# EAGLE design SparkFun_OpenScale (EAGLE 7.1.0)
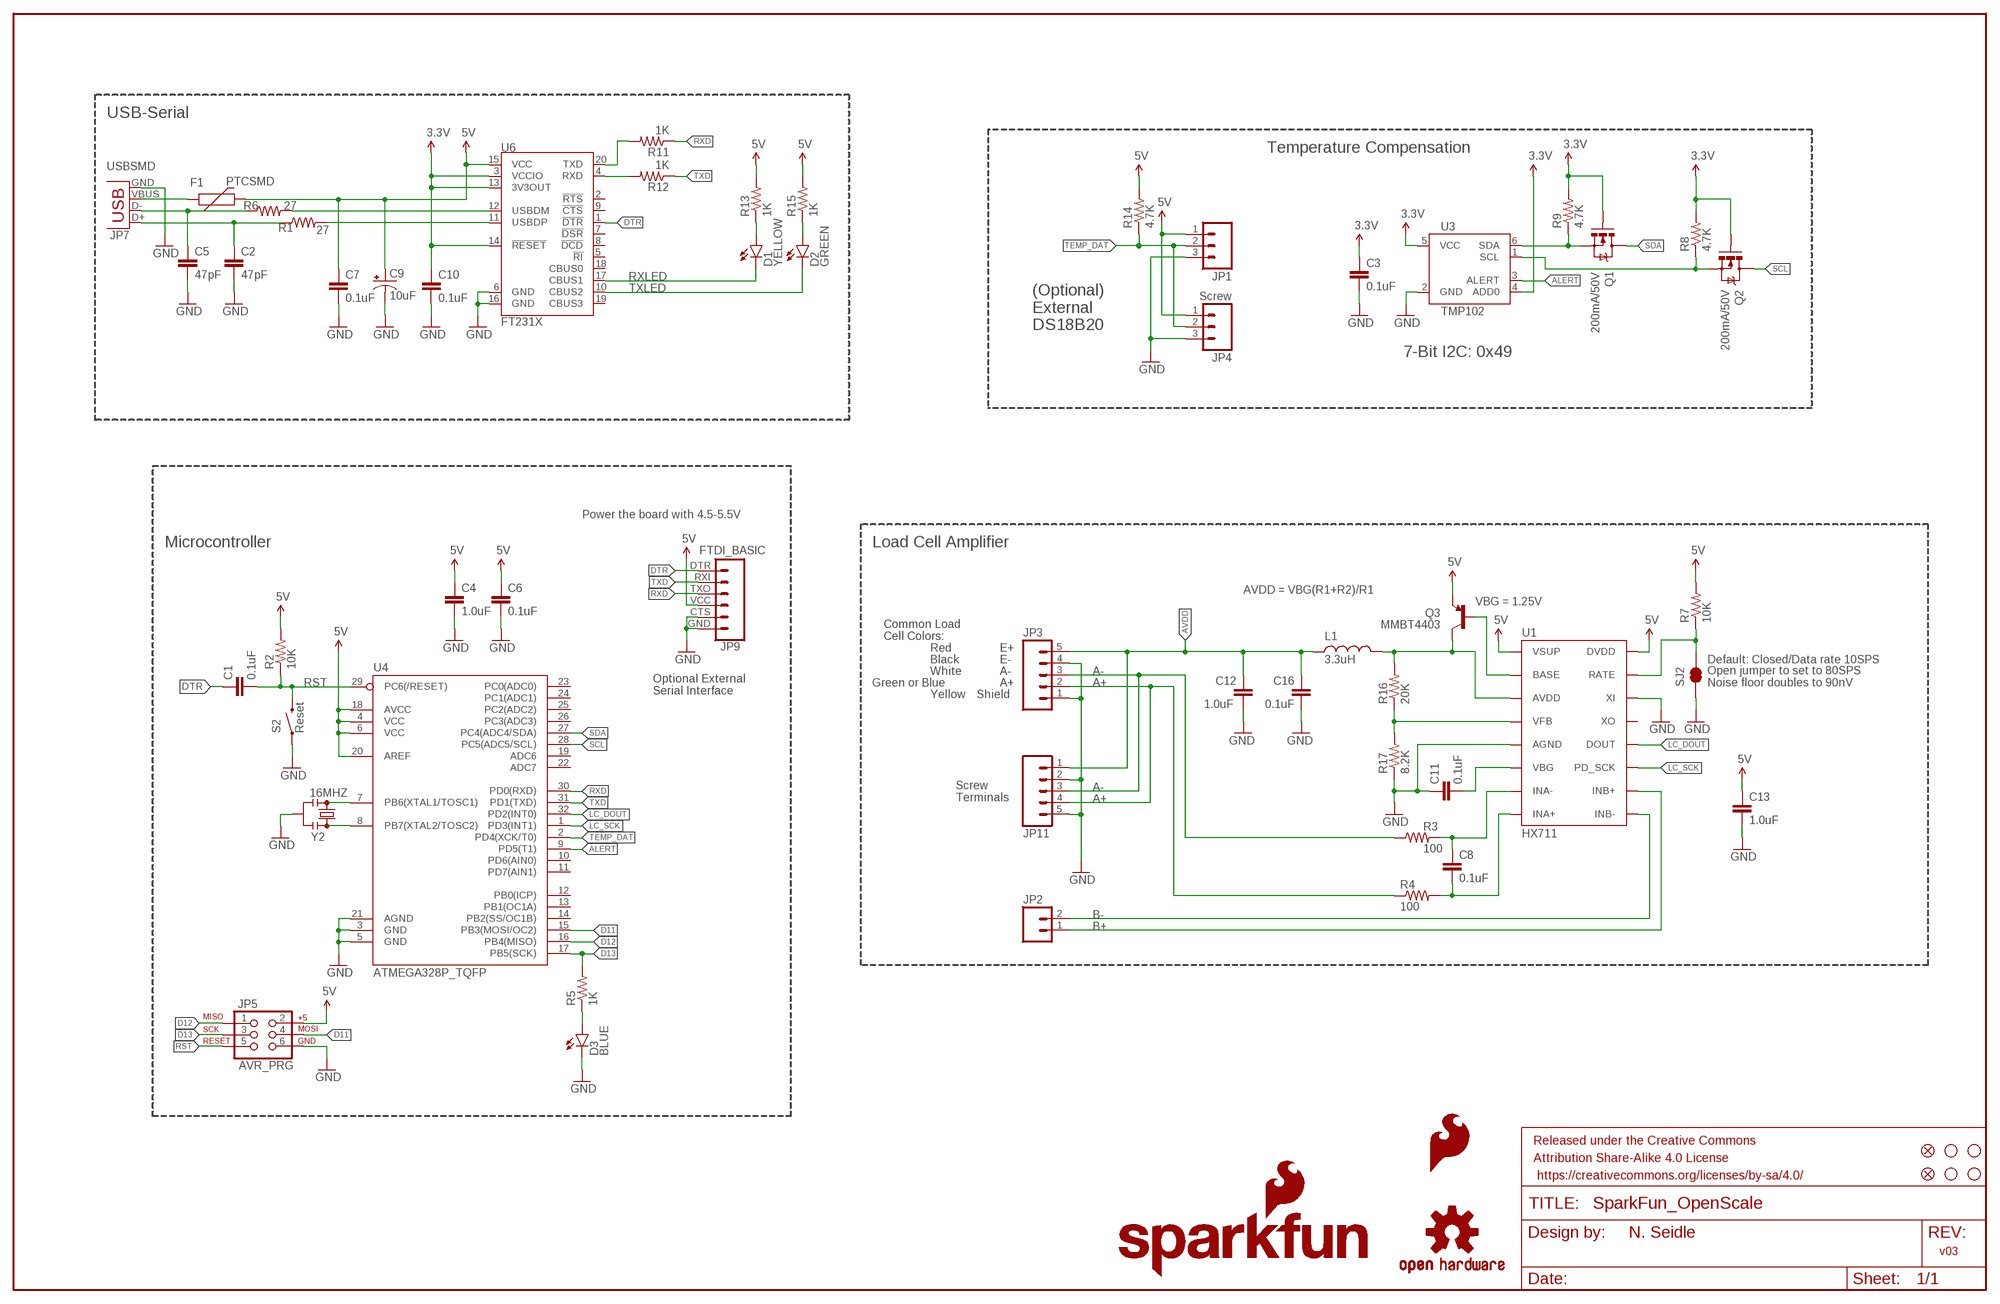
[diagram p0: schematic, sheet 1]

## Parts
C1  0.1uF  0.1UF-25V(+80/-20%)(0603)  [0603-CAP]
C2  47pF  47PF-50V-5%(0603)  [0603-CAP]
C3  0.1uF  0.1UF-25V(+80/-20%)(0603)  [0603-CAP]
C4  1.0uF  1.0UF-16V-10%(0603)  [0603-CAP]
C5  47pF  47PF-50V-5%(0603)  [0603-CAP]
C6  0.1uF  0.1UF-25V(+80/-20%)(0603)  [0603-CAP]
C7  0.1uF  0.1UF-25V(+80/-20%)(0603)  [0603-CAP]
C8  0.1uF  0.1UF-25V(+80/-20%)(0603)  [0603-CAP]
C9  10uF  10UF-16V-10%(TANT)  [EIA3216]
C10  0.1uF  0.1UF-25V(+80/-20%)(0603)  [0603-CAP]
C11  0.1uF  0.1UF-25V(+80/-20%)(0603)  [0603-CAP]
C12  1.0uF  1.0UF-16V-10%(0603)  [0603-CAP]
C13  1.0uF  1.0UF-16V-10%(0603)  [0603-CAP]
C16  0.1uF  0.1UF-25V(+80/-20%)(0603)  [0603-CAP]
D1  YELLOW  LED-YELLOWLARGE  [LED-1206]
D2  GREEN  LED-GREENLARGE  [LED-1206]
D3  BLUE  LED-BLUE1206  [LED-1206]
F1  PTCSMD  [PTC-1206]
FID1  FIDUCIAL1X2  [FIDUCIAL-1X2]
FID2  FIDUCIAL1X2  [FIDUCIAL-1X2]
FRAME1  FRAME-LEDGER  [CREATIVE_COMMONS]
JP1  M031X03_NO_SILK  [1X03_NO_SILK]
JP2  M02PTH  [1X02]
JP3  M05NO_SILK  [1X05_NO_SILK]
JP4  Screw  M03SCREW_LOCK  [SCREWTERMINAL-3.5MM-3_LOCK.007S]
JP5  AVR_PRG  AVR_SPI_PRG_6PTH  [2X3]
JP7  USBSMD  [USB-MINIB]
JP9  FTDI_BASIC  FTDI_BASICPTH  [FTDI_BASIC]
JP11  M05SCREW  [SCREWTERMINAL-3.5MM-5]
L1  3.3uH  INDUCTOR0805  [0805]
LOGO1  SFE_LOGO_NAME_FLAME.1_INCH  [SFE_LOGO_NAME_FLAME_.1]
LOGO2  OSHW-LOGOS  [OSHW-LOGO-S]
LOGO3  SFE_LOGO_FLAME.1_STOP  [SFE_LOGO_FLAME_STOP_.1]
LOGO4  SFE_LOGO_NAME_FLAME.1_INCH  [SFE_LOGO_NAME_FLAME_.1]
Q1  200mA/50V  MOSFET-NCHANNELBSS138  [SOT23-3]
Q2  200mA/50V  MOSFET-NCHANNELBSS138  [SOT23-3]
Q3  MMBT4403  TRANSISTOR_PNPMMBT4403  [SOT23-3]
R1  27  27OHM1/10W1%(0603)  [0603]
R2  10K  10KOHM-1/10W-1%(0603)0603  [0603-RES]
R3  100  100OHM-1/10W-1%(0603)  [0603-RES]
R4  100  100OHM-1/10W-1%(0603)  [0603-RES]
R5  1K  1KOHM-1/10W-1%(0603)  [0603-RES]
R6  27  27OHM1/10W1%(0603)  [0603]
R7  10K  10KOHM-1/10W-1%(0603)0603  [0603-RES]
R8  4.7K  4.7KOHM-1/10W-1%(0603)  [0603-RES]
R9  4.7K  4.7KOHM-1/10W-1%(0603)  [0603-RES]
R11  1K  1KOHM-1/10W-1%(0603)  [0603-RES]
R12  1K  1KOHM-1/10W-1%(0603)  [0603-RES]
R13  1K  1KOHM-1/10W-1%(0603)  [0603-RES]
R14  4.7K  4.7KOHM-1/10W-1%(0603)  [0603-RES]
R15  1K  1KOHM-1/10W-1%(0603)  [0603-RES]
R16  20K  20KOHM1/10W1%(0603)  [0603-RES]
R17  8.2K  8.2KOHM-1/10W-5%(0603)  [0603-RES]
S2  Reset  SWITCH-MOMENTARY-2SMD-1101NE  [TACTILE-SWITCH-1101NE]
SJ2  JUMPER-PAD-2-NC_BY_TRACE  [PAD-JUMPER-2-NC_BY_TRACE_YES_SILK]
STANDOFF1  STAND-OFF  [STAND-OFF]
STANDOFF2  STAND-OFF  [STAND-OFF]
STANDOFF3  STAND-OFF  [STAND-OFF]
STANDOFF4  STAND-OFF  [STAND-OFF]
U1  HX711  HX711HX711  [SO16]
U3  TMP102  [SOT563]
U4  ATMEGA328P_TQFP  [TQFP32-08]
U6  FT231X  FT231XS  [SSOP20_L]
Y2  16MHZ  RESONATOR16MHZ  [RESONATOR-SMD]

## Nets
3.3V [power]: C3.1 C10.1 Q1.1(G) Q2.1(G) R8.2 R9.2 U3.4(ADD0) U3.5(VCC) U6.3(VCCIO) U6.13(3V3OUT) U6.14(!RESET)
5V: C4.1 C6.1 C7.1 C9.A(+) C13.1 F1.2 JP1.1 JP4.1 JP5.2 JP9.VCC Q3.2(E) R2.2 R7.2 R13.2 R14.2 R15.2 U1.1(VSUP) U1.16(DVDD) U4.4(VCC) U4.6(VCC) U4.18(AVCC) U4.20(AREF) U6.15(VCC)
A+: JP3.2 JP11.4 R4.1
A-: JP3.3 JP11.3 R3.1
ALERT: U3.3(ALERT) U4.9(PD5(T1))
AVDD: C12.2 C16.1 JP3.5 JP11.1 L1.1
B+: JP2.1 U1.10(INB+)
B-: JP2.2 U1.9(INB-)
D11: JP5.4 U4.15(PB3(MOSI/OC2))
D12: JP5.1 U4.16(PB4(MISO))
D13: JP5.3 R5.2 U4.17(PB5(SCK))
DTR: C1.1 JP9.DTR U6.1(!DTR)
GND [power]: C2.2 C3.2 C4.2 C5.2 C6.2 C7.2 C9.C(-) C10.2 C11.1 C12.1 C13.2 C16.2 D3.C JP1.3 JP3.1 JP3.4 JP4.3 JP5.6 JP7.GND JP9.CTS JP9.GND JP11.2 JP11.5 R17.1 S2.1 SJ2.1 U1.5(AGND) U1.14(XI) U3.2(GND) U4.3(GND) U4.5(GND) U4.21(AGND) U6.6(GND) U6.16(GND) Y2.2
LC_DOUT: U1.12(DOUT) U4.32(PD2(INT0))
LC_SCK: U1.11(PD_SCK) U4.1(PD3(INT1))
LV_SCL: Q2.2(S) R8.1 U3.1(SCL)
LV_SDA: Q1.2(S) R9.1 U3.6(SDA)
N$1: U4.7(PB6(XTAL1/TOSC1)) Y2.1
N$2: D3.A R5.1
N$3: U4.8(PB7(XTAL2/TOSC2)) Y2.3
N$4: C5.1 JP7.D- R6.1
N$5: D1.A R13.1
N$6: D2.A R15.1
N$7: C2.1 JP7.D+ R1.1
N$8: R6.2 U6.12(USBDM)
N$9: R7.1 SJ2.2 U1.15(RATE)
N$10: C8.1 R3.2 U1.7(INA-)
N$11: C8.2 R4.2 U1.8(INA+)
N$12: F1.1 JP7.VBUS
N$13: R1.2 U6.11(USBDP)
N$14: R12.2 U6.4(RXD)
N$15: L1.2 Q3.3(C) R16.2 U1.3(AVDD)
N$16: R11.2 U6.20(TXD)
N$17: Q3.1(B) U1.2(BASE)
N$18: R16.1 R17.2 U1.4(VFB)
N$21: C11.2 U1.6(VBG)
RST: C1.2 JP5.5 R2.1 S2.2 U4.29(PC6(/RESET))
RXD: JP9.TXO R11.1 U4.30(PD0(RXD))
RXLED: D1.C U6.17(CBUS1)
SCL: Q2.3(D) U4.28(PC5(ADC5/SCL))
SDA: Q1.3(D) U4.27(PC4(ADC4/SDA))
TEMP_DAT: JP1.2 JP4.2 R14.1 U4.2(PD4(XCK/T0))
TXD: JP9.RXI R12.1 U4.31(PD1(TXD))
TXLED: D2.C U6.10(CBUS2)
Unconnected: U1.13(XO) U4.10(PD6(AIN0)) U4.11(PD7(AIN1)) U4.12(PB0(ICP)) U4.13(PB1(OC1A)) U4.14(PB2(SS/OC1B)) U4.19(ADC6) U4.22(ADC7) U4.23(PC0(ADC0)) U4.24(PC1(ADC1)) U4.25(PC2(ADC2)) U4.26(PC3(ADC3)) U6.2(!RTS) U6.5(!RI) U6.7(!DSR) U6.8(!DCD) U6.9(!CTS) U6.18(CBUS0) U6.19(CBUS3)

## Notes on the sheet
- USB-Serial
- Temperature Compensation
- (Optional)
  External
  DS18B20
- 7-Bit I2C: 0x49
- Power the board with 4.5-5.5V
- Microcontroller | Load Cell Amplifier
- AVDD = VBG(R1+R2)/R1
- VBG = 1.25V
- Common Load
  Cell Colors:
- Red | E+
- Black | E- | Default: Closed/Data rate 10SPS
- White | A-
- Green or Blue | A+
- Open jumper to set to 80SPS
  Noise floor doubles to 90nV
- Optional External
  Serial Interface
- Yellow | Shield
- Screw
  Terminals
- N. Seidle
- v03

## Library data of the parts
C1 C3 C6-C8 C10 C11 C16 = SparkFun-Capacitors:0.1UF-25V(+80/-20%)(0603): CAP-00810; PROD_ID: CAP-00810
C2 C5 = SparkFun-Capacitors:47PF-50V-5%(0603): CAP-08913; PROD_ID: CAP-08913
C4 C12 C13 = SparkFun-Capacitors:1.0UF-16V-10%(0603): CAP-00868; PROD_ID: CAP-00868
C9 = SparkFun-Capacitors:10UF-16V-10%(TANT): CAP-00811; PROD_ID: CAP-00811
D1 = SparkFun-LED:LED-YELLOW: Yellow SMD LEDs; PROD_ID: DIO-00820
D2 = SparkFun-LED:LED-GREEN: Various green LEDs; PROD_ID: DIO-00862
D3 = SparkFun-LED:LED-BLUE: Blue LEDs for production use; PROD_ID: DIO-09911
F1 = SparkFun-PowerIC:PTC: Resettable Fuse PTC; PROD_ID: RES-11150
FID1 FID2 = SparkFun-Aesthetics:FIDUCIAL: Fiducial Alignment Points
FRAME1 = SparkFun-Aesthetics:FRAME-LEDGER: Schematic Frame; DESIGNER: N. Seidle; VERSION: v02
JP1 = SparkFun-Connectors:M03: Header 3 Standard 3-pin 0.1" header. Use with straight break away headers (SKU : PRT-00116), right angle break away headers (PRT-00553), swiss pins (PRT-00743), machine pins (PRT-00117), and female headers (PRT-00115). Molex polarized connector foot print use with SKU : PRT-08232 with associated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
JP2 = SparkFun-Connectors:M02: Standard 2-pin 0.1" header. Use with
JP3 = SparkFun-Connectors:M05: Header 5 Standard 5-pin 0.1" header. Use with straight break away headers (SKU : PRT-00116), right angle break away headers (PRT-00553), swiss pins (PRT-00743), machine pins (PRT-00117), and female headers (PRT-00115). Molex polarized connector foot print use with SKU : PRT-08230 with associated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
JP4 = SparkFun-Connectors:M03: Header 3 Standard 3-pin 0.1" header. Use with straight break away headers (SKU : PRT-00116), right angle break away headers (PRT-00553), swiss pins (PRT-00743), machine pins (PRT-00117), and female headers (PRT-00115). Molex polarized connector foot print use with SKU : PRT-08232 with associated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; PROD_ID: CONN-08288
JP5 = SparkFun-Connectors:AVR_SPI_PRG_6: AVR ISP 6 Pin This is the reduced ISP connector for AVR programming. Common on Arduino. This footprint will take up less PCB space and can be used with a 10-pin to 6-pin adapter such as SKU: BOB-08508 **Special note about "TEST_POINT" package. The stop mask is on the top side, so if you want your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
JP7 = SparkFun-Connectors:USB: USB Connectors USB-B-PTH is fully proven SKU : PRT-00139/CONN-08278 USB-miniB is fully proven SKU : PRT-00587 USB-A-PCB is untested. USB-A-H is throughly reviewed, but untested. Spark Fun Electronics SKU : PRT-00437 USB-B-SMT is throughly reviewed, but untested. Needs silkscreen touching up.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; PROD_ID: CONN-08193
JP9 = SparkFun-Connectors:FTDI_BASIC: FTDI Basic header with labels
JP11 = SparkFun-Connectors:M05: Header 5 Standard 5-pin 0.1" header. Use with straight break away headers (SKU : PRT-00116), right angle break away headers (PRT-00553), swiss pins (PRT-00743), machine pins (PRT-00117), and female headers (PRT-00115). Molex polarized connector foot print use with SKU : PRT-08230 with associated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; PROD_ID: Combine 8288+8399
L1 = SparkFun-Passives:INDUCTOR: Inductors
LOGO1 LOGO4 = SparkFun-Aesthetics:SFE_LOGO_NAME_FLAME: SFE Logo, name and flame
LOGO2 = SparkFun-Aesthetics:OSHW-LOGO: Open Source Hardware Logo
LOGO3 = SparkFun-Aesthetics:SFE_LOGO_FLAME: SFE Logo, flame only
Q1 Q2 = SparkFun-DiscreteSemi:MOSFET-NCHANNEL: Common NMOSFET Parts MFG P/NStore IDProd ID FDD8780TRANS-09984 SI7820DNTRANS-11055 FDS6630AIC-08089 2N7002PWTRANS-11151 FQP30N06L COM-10213TRANS-10060 BSS123LT1GTRANS-08345 BSS138TRANS-00830 BS170 2N7000; PROD_ID: TRANS-00830
Q3 = SparkFun-DiscreteSemi:TRANSISTOR_PNP: Generic PNP BJT Double check pinouts against datasheets- not all devices are the same! MMBT3906 - 40V 200mA SOT-23 (TRANS-08052) MMBT4403 - 40V 600mA SOT-23 (TRANS-09245); PROD_ID: TRANS-09245
R1 R6 = SparkFun-Resistors:27OHM1/10W1%(0603): RES-09334; PROD_ID: RES-09334
R2 R7 = SparkFun-Resistors:10KOHM-1/10W-1%(0603): RES-00824; PROD_ID: RES-00824
R3 R4 = SparkFun-Resistors:100OHM-1/10W-1%(0603): RES-07863; PROD_ID: RES-07863
R5 R11-R13 R15 = SparkFun-Resistors:1KOHM-1/10W-1%(0603): RES-07856; PROD_ID: RES-07856
R8 R9 R14 = SparkFun-Resistors:4.7KOHM-1/10W-1%(0603): RES-07857; PROD_ID: RES-07857
R16 = SparkFun-Resistors:20KOHM1/10W1%(0603): RES-09383; PROD_ID: RES-09383; VALUE: 20k
R17 = SparkFun-Resistors:8.2KOHM-1/10W-5%(0603): RES-10646; PROD_ID: RES-10646
S2 = SparkFun-Electromechanical:SWITCH-MOMENTARY-2: Various NO switches- pushbuttons, reed, etc; PROD_ID: SWCH-00815
SJ2 = SparkFun-Passives:JUMPER-PAD-2-NC_BY_TRACE
STANDOFF1-STANDOFF4 = SparkFun-Electromechanical:STAND-OFF: #4 Stand Off
U1 = Testing:HX711; PROD_ID: IC-12445
U3 = SparkFun-Sensors:TMP102: I2C degC temp sensor; PROD_ID: IC-09303
U4 = SparkFun-DigitalIC:ATMEGA328P_TQFP; PROD_ID: IC-09069
U6 = SparkFun-DigitalIC:FT231X: FTDI FT231X Full Speed USB to Full-handshake UART This USB2.0 Full Speed IC offers a compact bridge to full handshake UART interfaces. The device is a UART, capable of operating up to 3MBaud, with low power consumption (8mA). The FT231X includes the complete FT-X series feature set and enables USB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; PROD_ID: IC-11524; VALUE: FTS31XS-U
Y2 = SparkFun-FreqCtrl:RESONATOR: Resonator Small SMD resonator. Used, eg, on the Arduino Pro/ Pro Mini boards. 8MHz- XTAL-08895 16MHz- XTAL-08900; PROD_ID: XTAL-08900

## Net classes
1 power: width 0.203 mm

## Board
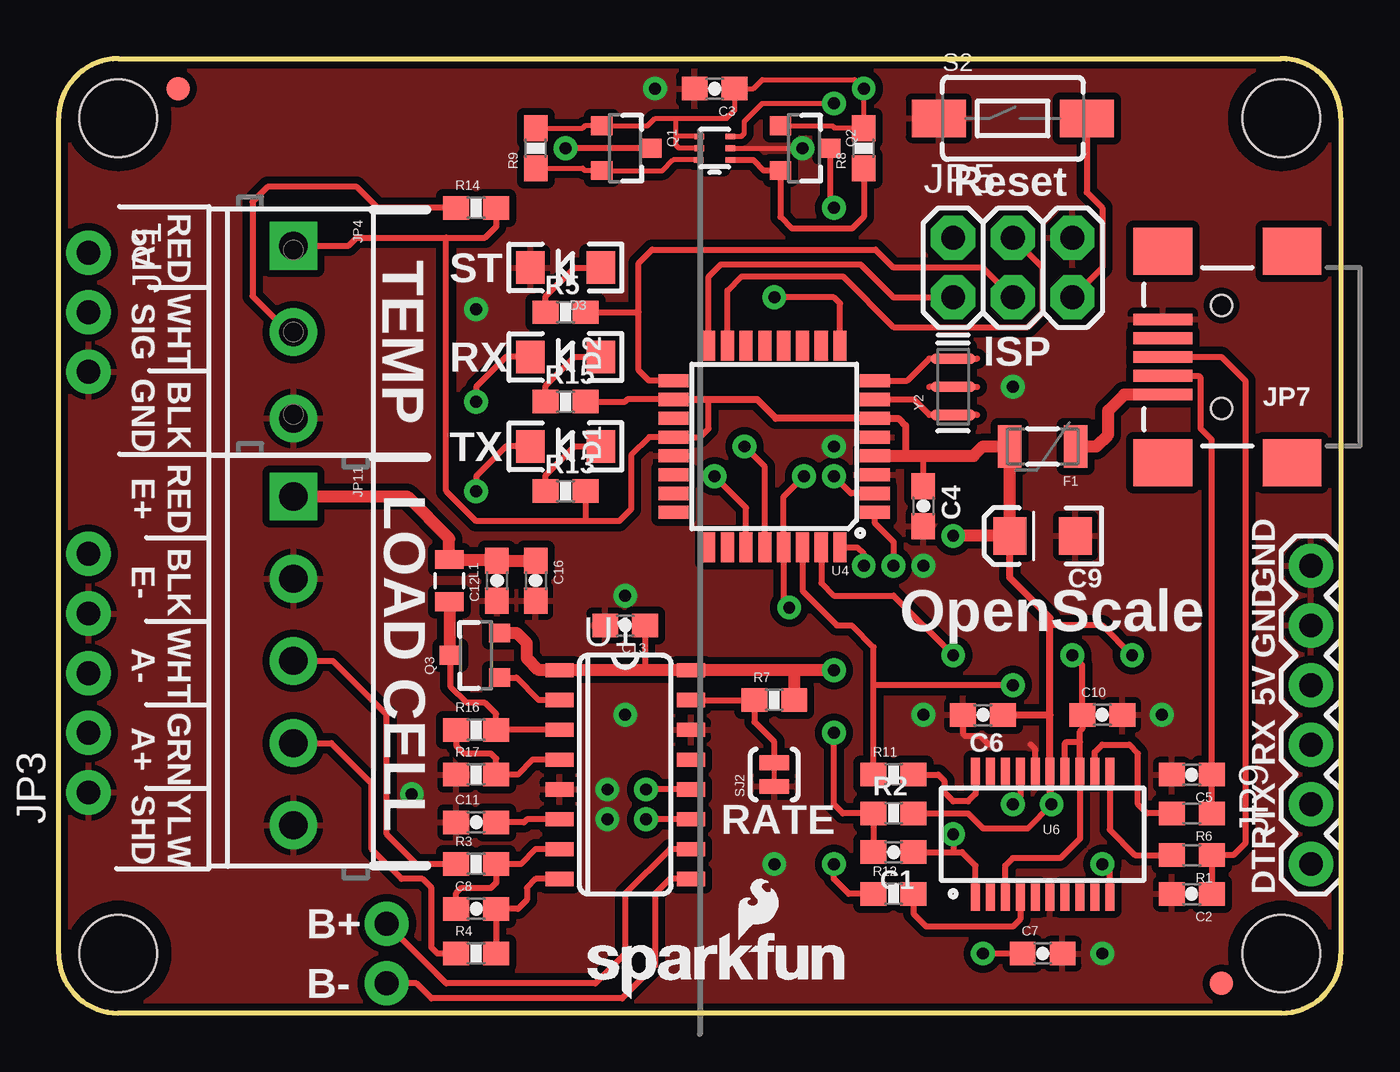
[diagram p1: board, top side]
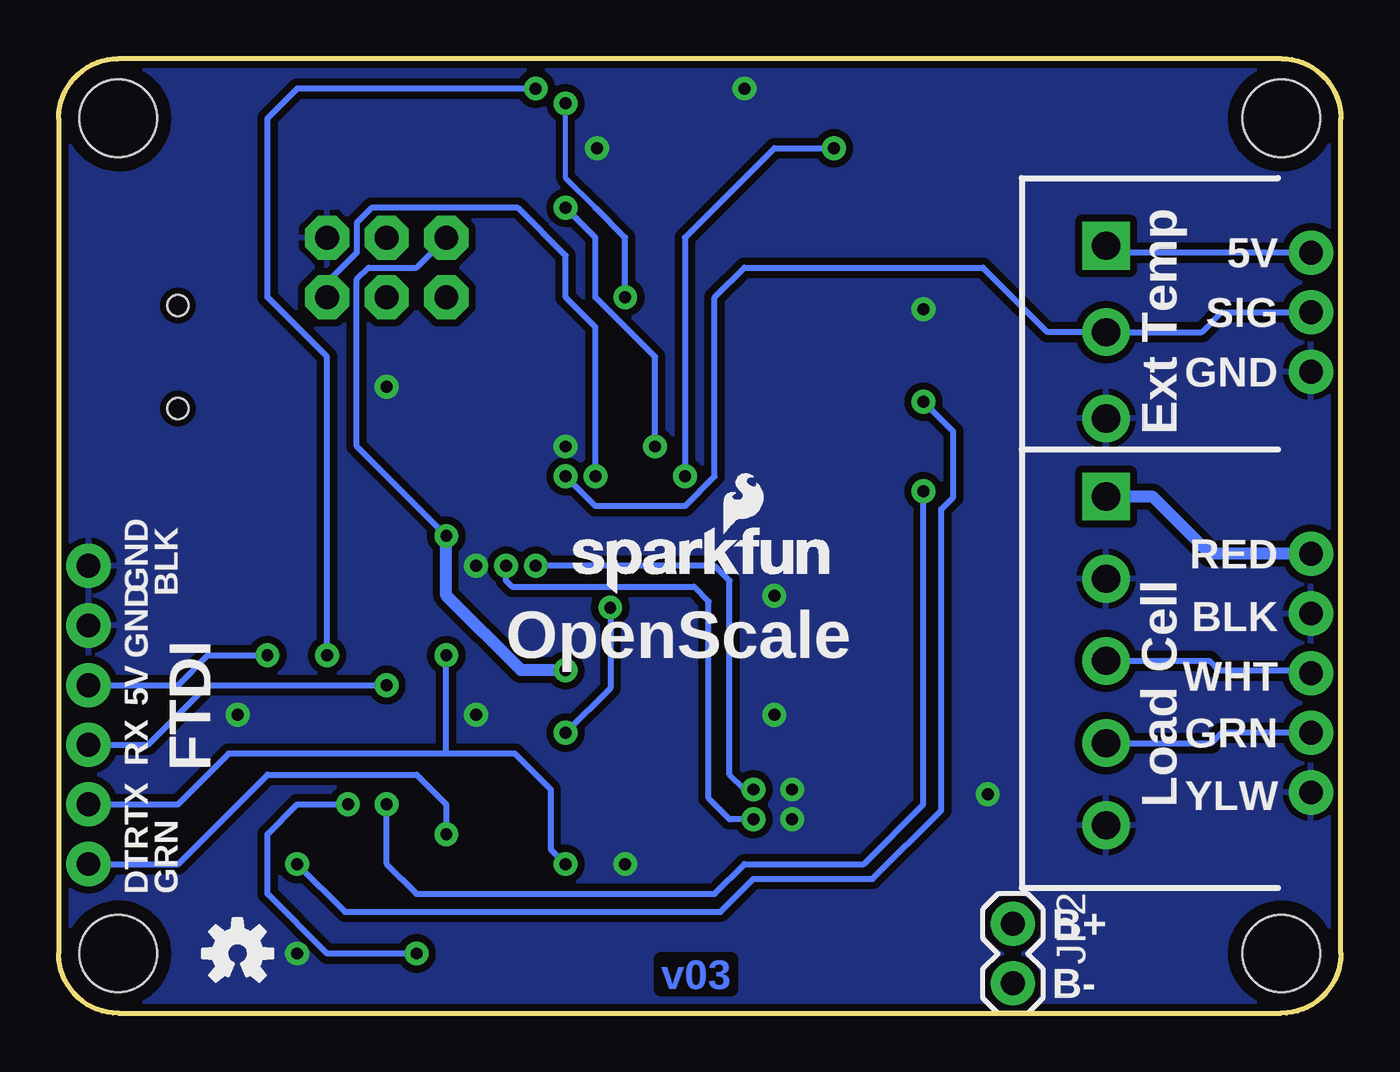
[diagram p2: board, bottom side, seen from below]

Size 54.61 x 40.64 mm. Coordinates in mm from the lower left corner, seen from the top.
Outline: 52.07,0 2.54,0 arc-90 0,2.54 0,38.1 arc-90 2.54,40.64 52.07,40.64 arc-90 54.61,38.1 54.61,2.54 arc-90 52.07,0
Copper layers (1*16): Top 0.035mm / dielectric 1.5mm / Bottom 0.035mm
Design rules "SparkFun-2-layer *": minimum track width 7mil, minimum drill 15mil, track to track 8mil, track to pad 8mil, pad to pad 8mil, via to via 8mil, smd to smd 8mil, copper to edge 8mil, drill to drill 8mil, minimum pad ring 12mil, minimum via ring 10mil, stop-mask expansion 4mil, vias tented up to drill 20mil, thermal gap 10mil
tRestrict: area 27.6,35.9 to 28.3,37.7

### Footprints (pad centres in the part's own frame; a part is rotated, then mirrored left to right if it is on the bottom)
0603-CAP = smd 1.1 x 1: 1 -0.85,0; 2 0.85,0
EIA3216 = smd 1.4 x 1.6: A 1.4,0; C -1.4,0
LED-1206 = smd 1.2 x 1.4: A -1.5,0; C 1.5,0
PTC-1206 = smd 1 x 1.8: 1 -1.4,0; 2 1.4,0
FIDUCIAL-1X2 = smd 1 x 1: 1 0,0
1X03_NO_SILK = drill 1.016 pad 1.88: 1 0,0; 2 2.54,0; 3 5.08,0
1X02 = drill 1.016 pad 1.88: 1 0,0; 2 2.54,0
1X05_NO_SILK = drill 1.016 pad 1.88: 1 0,0; 2 2.54,0; 3 5.08,0; 4 7.62,0; 5 10.16,0
SCREWTERMINAL-3.5MM-3_LOCK.007S = drill 1.2 pad 2.032 square: 1 -0.178,0 | drill 1.2 pad 2.032: 2 3.5,0; 3 7.178,0
2X3 = drill 1.016 pad 1.88 octagon: 1 0,0; 2 0,2.54; 3 2.54,0; 4 2.54,2.54; 5 5.08,0; 6 5.08,2.54
USB-MINIB = smd 2.5 x 0.5: D+ 2.5,0; D- 2.5,0.8; GND 2.5,-1.6; ID 2.5,-0.8; VBUS 2.5,1.6 | smd 2.5 x 2: MTN1 -3,4.5; MTN2 2.5,4.5; MTN3 -3,-4.5; MTN4 2.5,-4.5 | hole 0.9: 0,2.2; 0,-2.2
FTDI_BASIC = drill 1.016 pad 1.88: CTS 10.16,0; DTR 0,0; GND 12.7,0; RXI 2.54,0; TXO 5.08,0; VCC 7.62,0
SCREWTERMINAL-3.5MM-5 = drill 1.2 pad 2.032 square: 1 0,0 | drill 1.2 pad 2.032: 2 3.5,0; 3 7,0; 4 10.5,0; 5 14,0
0805 = smd 0.8 x 1.2: 1 -0.9,0; 2 0.9,0
SOT23-3 = smd 0.8 x 0.9: 1 -0.95,-1; 2 0.95,-1; 3 0,1.1
0603 = smd 1.1 x 1: 1 -0.85,0; 2 0.85,0
0603-RES = smd 1.1 x 1: 1 -0.85,0; 2 0.85,0
TACTILE-SWITCH-1101NE = smd 2.3 x 1.6: 1 -3.15,0; 2 3.15,0
PAD-JUMPER-2-NC_BY_TRACE_YES_SILK = smd 0.635 x 1.27: 1 -0.508,0; 2 0.508,0
STAND-OFF = hole 3.302: 0,0
SO16 = smd 0.6 x 1.2: 1 -4.445,-2.8; 2 -3.175,-2.8; 3 -1.905,-2.8; 4 -0.635,-2.8; 5 0.635,-2.8; 6 1.905,-2.8; 7 3.175,-2.8; 8 4.445,-2.8; 9 4.445,2.8; 10 3.175,2.8; 11 1.905,2.8; 12 0.635,2.8; 13 -0.635,2.8; 14 -1.905,2.8; 15 -3.175,2.8; 16 -4.445,2.8
SOT563 = smd 0.25 x 0.4: 1 -0.5,-0.66; 2 0,-0.66; 3 0.5,-0.66; 4 0.5,0.66; 5 0,0.66; 6 -0.5,0.67
TQFP32-08 = smd 1.27 x 0.559: 1 -4.293,2.8; 2 -4.293,2; 3 -4.293,1.2; 4 -4.293,0.4; 5 -4.293,-0.4; 6 -4.293,-1.2; 7 -4.293,-2; 8 -4.293,-2.8; 17 4.293,-2.8; 18 4.293,-2; 19 4.293,-1.2; 20 4.293,-0.4; 21 4.293,0.4; 22 4.293,1.2; 23 4.293,2; 24 4.293,2.8 | smd 0.559 x 1.27: 9 -2.8,-4.293; 10 -2,-4.293; 11 -1.2,-4.293; 12 -0.4,-4.293; 13 0.4,-4.293; 14 1.2,-4.293; 15 2,-4.293; 16 2.8,-4.293; 25 2.8,4.293; 26 2,4.293; 27 1.2,4.293; 28 0.4,4.293; 29 -0.4,4.293; 30 -1.2,4.293; 31 -2,4.293; 32 -2.8,4.293
SSOP20_L = smd 0.381 x 1.143: 1 -2.857,-2.68; 2 -2.223,-2.68; 3 -1.587,-2.68; 4 -0.953,-2.68; 5 -0.318,-2.68; 6 0.318,-2.68; 7 0.953,-2.68; 8 1.587,-2.68; 9 2.223,-2.68; 10 2.857,-2.68; 11 2.857,2.68; 12 2.223,2.68; 13 1.587,2.68; 14 0.953,2.68; 15 0.318,2.68; 16 -0.318,2.68; 17 -0.953,2.68; 18 -1.587,2.68; 19 -2.223,2.68; 20 -2.857,2.68
RESONATOR-SMD = smd 0.45 x 1.905: 1 -1.2,0; 2 0,0; 3 1.2,0

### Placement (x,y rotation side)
C1  35.56,6.86 180 top
C2  48.26,5.08 180 top
C3  27.94,39.37 180 top
C4  36.83,21.59 270 top
C5  48.26,10.16 180 top
C6  39.37,12.7 180 top
C7  41.91,2.54 0 top
C8  17.78,4.45 0 top
C9  41.91,20.32 180 top
C10  44.45,12.7 0 top
C11  17.78,8.13 0 top
C12  18.67,18.41 90 top
C13  24.13,16.51 180 top
C16  20.32,18.41 270 top
D1  21.59,24.13 180 top
D2  21.59,27.94 180 top
D3  21.59,31.75 180 top
F1  41.91,24.13 180 top
FID1  49.53,1.27 0 top
FID2  5.08,39.37 0 top
FRAME1  not placed on the board
JP1  1.27,32.38 270 top
JP2  13.97,3.81 270 bottom
JP3  1.27,9.4 90 top
JP4  10,32.5 270 top
JP5  38.1,30.48 0 top
JP7  49.53,27.94 180 top
JP9  53.34,6.35 90 top
JP11  10,22 270 top
L1  16.64,18.41 270 top
LOGO1  22.1,0.51 0 top
LOGO2  46.99,2.54 0 bottom
LOGO3  46.48,35.18 0 top
LOGO4  33.15,17.78 0 bottom
Q1  24.13,36.83 270 top
Q2  31.75,36.83 270 top
Q3  17.78,15.24 90 top
R1  48.26,6.73 180 top
R2  35.56,8.51 0 top
R3  17.78,6.35 0 top
R4  17.78,2.54 0 top
R5  21.59,29.84 0 top
R6  48.26,8.51 180 top
R7  30.48,13.34 0 top
R8  34.29,36.83 90 top
R9  20.32,36.83 90 top
R11  35.56,10.16 0 top
R12  35.56,5.08 0 top
R13  21.59,22.23 0 top
R14  17.78,34.29 0 top
R15  21.59,26.04 0 top
R16  17.78,12.06 0 top
R17  17.78,10.16 0 top
S2  40.64,38.1 0 top
SJ2  30.48,10.16 90 top
STANDOFF1  52.07,38.1 0 top
STANDOFF2  52.07,2.54 0 top
STANDOFF3  2.54,2.54 0 top
STANDOFF4  2.54,38.1 0 top
U1  24.13,10.16 270 top
U3  27.94,36.83 90 top
U4  30.48,24.13 180 top
U6  41.91,7.62 0 top
Y2  38.1,26.67 90 top

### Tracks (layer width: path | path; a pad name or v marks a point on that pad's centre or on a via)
3.3V  (via drill 0.51)
  Top 0.203: U3.5 26.42,36.83 26.29,36.96 26.29,37.34 | 26.29,37.34 26.29,38.1 | U3.4 26.3,37.33 26.29,37.34 | R9.2 22.31,37.68 22.41,37.78 Q1.1 25.08,37.78 25.4,38.1 26.29,38.1 | Q2.1 32.96,37.78 33.06,37.68 R8.2 v34.29,39.37 33.91,39.75 29.97,39.75 29.59,39.37 C3.1 28.79,38.44 28.45,38.1 26.29,38.1
  Top 0.254: U6.14 42.86,11.49 42.93,11.56 43.5,11.56 | v43.18,15.24 43.6,14.82 C10.1 43.6,12.1 43.5,12 43.5,11.56 | U6.3 40.32,6.29 40.64,6.6 42.67,6.6 43.5,7.43 U6.13 43.5,11.56
  Bottom 0.254: v43.18,15.24 43.18,27.94 45.72,30.48 45.72,38.1 44.45,39.37 v34.29,39.37
5V  (via drill 0.51)
  Top 0.254: 22.54,26.13 R15.2 24.13,26.04 24.23,26.13 U4.18 | 27.69,26.13 27.69,24.89 27.32,24.53 U4.20 25.16,24.53 24.38,23.75 24.38,21.46 23.88,20.95 22.48,20.95 | C4.1 36.83,23.73 | R13.2 22.44,20.99 22.48,20.95 | C7.1 v39.37,2.54 | R2.2 38.73,8.51 39.37,7.87 41.27,7.87 v42.29,8.89 42.23,8.95 42.23,9.34 | v45.72,15.24 44.45,16.51 42.23,16.51 | 22.48,20.95 17.78,20.95 16.51,22.23 16.51,33.02 | 16.51,33.02 12.7,33.02 12.36,32.68 JP4.1 | 16.51,33.02 18.16,33.02 18.63,33.49 R14.2 | C13.1 24.98,14.69 24.89,14.61
  Top 0.305: 36.07,23.73 36.07,25.02 35.76,25.33 U4.6 30.55,25.33 29.75,26.13 27.69,26.13 U4.18 | 42.23,12.7 U6.15 42.23,9.34 | 42.23,12.7 42.23,16.51 42.23,16.83 40.51,18.55 C9.A | C6.1 42.23,12.7
  Top 0.508: U4.4 36.07,23.73 36.83,23.73 38.97,23.73 39.37,24.13 F1.2 C9.A v38.1,20.32 | v33.02,14.61 31.24,14.61 | 31.24,14.61 U1.16 24.89,14.61 U1.1 20.45,14.61 19.94,15.11 19.94,15.75 19.5,16.19 Q3.2 | R7.2 31.33,14.52 31.24,14.61
  Bottom 0.254: v39.37,2.54 43.18,2.54 45.72,5.08 45.72,7.62 44.45,8.89 v42.29,8.89 | JP9.VCC 49.53,13.97 48.26,15.24 v45.72,15.24 | v38.1,20.32 41.91,24.13 41.91,31.24 41.4,31.75 39.37,31.75 JP5.2 | JP1.1 9.71,32.38 JP4.1
  Bottom 0.508: v33.02,14.61 34.92,14.61 38.1,17.78 v38.1,20.32
A+
  Top 0.254: R4.1 16.13,2.54 15.88,2.79 15.88,5.33 15.49,5.71 14.61,5.71 13.34,6.99 13.34,9.78 11.61,11.5 JP11.4
  Bottom 0.254: JP3.2 5.08,11.94 5.52,11.5 JP11.4
A-
  Top 0.254: R3.1 15.24,6.35 13.97,7.62 13.97,12.7 11.67,15 JP11.3
  Bottom 0.254: JP3.3 1.38,14.59 5.19,14.59 5.6,15 JP11.3
ALERT  (via drill 0.51)
  Top 0.203: U3.3 29.07,37.33 29.21,37.47 29.21,37.97 29.97,38.73 v33.02,38.73
  Top 0.254: U4.9 33.28,30.22 33.02,30.48 v30.48,30.48
  Bottom 0.203: 31.75,34.29 33.02,35.56 v33.02,38.73
  Bottom 0.254: v30.48,30.48 30.48,33.02 31.75,34.29
AVDD
  Top 0.508: JP11.1 14.83,22 16.64,20.19 L1.1 18.62,19.32 C12.2 C16.1
  Bottom 0.508: JP3.5 5.59,19.56 8.03,22 JP11.1
B+
  Top 0.254: U1.10 26.04,6.99 24.13,5.08 24.13,2.54 22.86,1.27 16.51,1.27 JP2.1
B-
  Top 0.254: U1.9 26.04,5.71 25.4,5.08 25.4,2.03 24,0.64 15.88,0.64 15.24,1.27 JP2.2
D11
  Top 0.254: JP5.4 41.91,31.75 41.91,29.84 41.27,29.21 35.56,29.21 33.4,31.37 29.08,31.37 28.48,30.77 U4.15
D12
  Top 0.254: JP5.1 35.56,30.48 34.16,31.88 28.19,31.88 27.68,31.36 U4.16
D13
  Top 0.254: 24.7,29.84 24.7,27.37 25.14,26.93 U4.17 | R5.2 24.7,29.84 | JP5.3 39.37,31.75 35.56,31.75 34.8,32.51 25.27,32.51 24.7,31.94 24.7,29.84
DTR  (via drill 0.51)
  Top 0.254: U6.1 39.05,6.29 38.48,6.86 38.1,6.86 | C1.1 38.1,6.86 | v38.1,7.62 38.1,6.86
  Bottom 0.254: JP9.DTR 49.53,6.35 45.72,10.16 39.37,10.16 38.1,8.89 v38.1,7.62
GND  (via drill 0.51)
  Top 0.203: U3.2 v31.67,36.83
  Top 0.254: U6.16 41.59,11.24 41.4,11.43 | C6.2 38.52,11.9 38.61,11.81 39.24,11.81 39.62,11.43
  other vias: 17.78,29.97 24.13,17.78 23.37,9.53 23.37,8.26 15.04,9.32 30.48,6.35 33.02,24.13 36.83,19.05 46.99,12.7 44.45,2.54 36.83,12.7 40.64,26.67 24.13,12.7 25.4,39.37
  pour Top (isolate 0.305, rank 6): 55.88,40.64 0,40.64 0,0 55.88,0
  pour Bottom (isolate 0.305, rank 6): 55.88,40.64 0,40.64 0,0 55.88,0
LC_DOUT  (via drill 0.51)
  Top 0.254: v34.29,19.05 34.29,19.56 34.01,19.84 U4.32 | U1.12 v25.02,9.53
  Bottom 0.254: v34.29,19.05 26.67,19.05 26.04,18.41 26.04,10.16 25.4,9.53 v25.02,9.53
LC_SCK  (via drill 0.51)
  Top 0.254: v35.56,19.05 35.56,20.07 34.77,20.85 U4.1 | U1.11 v25.02,8.26
  Bottom 0.254: v35.56,19.05 35.56,18.41 35.31,18.16 27.56,18.16 26.92,17.53 26.92,9.14 26.04,8.26 v25.02,8.26
LV_SCL
  Top 0.254: U3.1 29.58,36.33 30.03,35.88 Q2.2 30.75,33.92 30.73,33.91 31.24,33.4 33.78,33.4 34.29,33.91 R8.1
LV_SDA
  Top 0.203: U3.6 26.17,36.33 25.72,35.88 Q1.2 22.41,35.88 22.31,35.98 R9.1
N$1
  Top 0.254: U4.7 36.42,26.13 37.08,25.47
N$2
  Top 0.254: R5.1 20.74,30.52 21.97,31.75 D3.A
N$3
  Top 0.254: U4.8 36.14,26.93 37.08,27.87
N$4
  Top 0.254: R6.1 C5.1 49.11,24.42 48.64,24.89 48.64,27.05 48.55,27.14 JP7.D-
N$5
  Top 0.254: R13.1 20.74,22.9 21.97,24.13 D1.A
N$6
  Top 0.254: R15.1 20.74,26.71 21.97,27.94 D2.A
N$7
  Top 0.254: C2.1 R1.1 50.04,6.73 50.55,7.24 50.55,26.92 49.53,27.94 JP7.D+
N$8
  Top 0.254: R6.2 46.35,8.51 45.97,8.89 45.97,11.05 45.59,11.43 44.45,11.43 44.13,11.11 U6.12
N$9
  Top 0.254: U1.15 R7.1 29.63,12.41 30.48,11.56 SJ2.2
N$10
  Top 0.254: C8.1 16.93,5.12 17.14,5.33 18.41,5.33 18.63,5.55 R3.2 19.68,6.35 20.32,6.99 U1.7
N$11
  Top 0.254: R4.2 C8.2 19.56,4.45 19.94,4.83 19.94,5.33 20.32,5.71 U1.8
N$12
  Top 0.508: JP7.VBUS 45.39,26.34 44.7,25.65 44.7,24.64 44.2,24.13 F1.1
N$13
  Top 0.254: U6.11 44.77,7.81 45.85,6.73 R1.2
N$14
  Top 0.254: U6.4 40.96,4 40.64,3.68 36.96,3.68 36.41,4.23 R12.2
N$15
  Top 0.254: U1.3 R16.2 18.63,12.74 18.16,13.21 17.4,13.21 16.68,13.93 Q3.3 | 16.68,17.43 16.68,17.47 L1.2
  Top 0.508: Q3.3 16.68,17.43
N$16
  Top 0.254: U6.20 39.05,9.34 38.73,9.02 38.1,9.02 37.72,9.4 37.72,9.91 37.47,10.16 R11.2
N$17
  Top 0.254: U1.2 20.45,13.34 19.49,14.29 Q3.1
N$18
  Top 0.254: R16.1 16.93,11.39 17.27,11.05 18.41,11.05 18.63,10.83 R17.2 19.56,10.16 20.19,10.79 U1.4
N$21
  Top 0.254: U1.6 19.94,8.26 19.81,8.13 C11.2
RST  (via drill 0.51)
  Top 0.254: v31.75,22.86 30.88,21.99 U4.29 30.88,17.51 v31.11,17.27 | C1.2 R2.1 33.4,8.51 33.02,8.89 v33.02,11.94 | S2.2 43.79,34.95 44.45,34.29 44.45,31.75 JP5.5
  Bottom 0.254: v31.75,22.86 31.75,29.21 33.02,30.48 33.02,32.26 35.05,34.29 41.27,34.29 41.91,33.66 41.91,32.38 43.18,31.11 JP5.5 | v33.02,11.94 31.11,13.84 v31.11,17.27
RXD  (via drill 0.51)
  Top 0.254: U4.30 31.68,17.98 33.15,16.51 33.78,16.51 34.71,15.58 34.71,13.97 | v40.64,13.97 34.71,13.97 | R11.1 34.71,13.97
  Bottom 0.254: JP9.TXO 50.8,11.43 48.26,13.97 v40.64,13.97
RXLED  (via drill 0.51)
  Top 0.254: D1.C 19.05,24.13 17.78,22.86 v17.78,22.23 | U6.17 40.96,9.21 v40.64,8.89
  Bottom 0.254: v40.64,8.89 40.64,6.35 39.37,5.08 26.67,5.08 25.4,6.35 20.32,6.35 17.78,8.89 v17.78,22.23
SCL  (via drill 0.51)
  Top 0.254: v29.21,24.13 30.08,23.26 U4.28 | Q2.3 32.85,34.46 v33.02,34.29
  Bottom 0.254: v33.02,34.29 31.75,33.02 31.75,30.48 29.21,27.94 v29.21,24.13
SDA  (via drill 0.51)
  Top 0.254: v27.94,22.86 29.28,21.52 U4.27 | Q1.3 v21.59,36.83
  Bottom 0.254: v27.94,22.86 27.94,33.02 24.13,36.83 v21.59,36.83
TEMP_DAT  (via drill 0.51)
  Top 0.254: v33.02,22.86 33.75,22.13 U4.2 | R14.1 13.59,34.29 12.7,35.18 8.89,35.18 8.26,34.54 8.26,30.54 9.79,29 JP4.2
  Bottom 0.254: v33.02,22.86 31.75,21.59 27.94,21.59 26.67,22.86 26.67,30.48 25.4,31.75 15.24,31.75 12.49,29 JP4.2 5.92,29 5.08,29.84 JP1.2
TXD  (via drill 0.51)
  Top 0.254: U4.31 32.48,18.32 33.02,17.78 35.56,17.78 v38.1,15.24 | R12.1 33.66,5.08 33.02,5.71 v33.02,6.35
  Bottom 0.254: v33.02,6.35 33.66,6.99 33.66,9.53 35.18,11.05 38.1,11.05 | 38.1,11.05 v38.1,15.24 | JP9.RXI 49.53,8.89 47.37,11.05 38.1,11.05
TXLED  (via drill 0.51)
  Top 0.254: D2.C 19.05,27.94 17.78,26.67 v17.78,26.04 | U6.10 44.77,6.03 v44.45,6.35
  Bottom 0.254: v17.78,26.04 16.51,24.77 16.51,21.97 17.02,21.46 17.02,8.64 19.94,5.71 25.02,5.71 26.42,4.32 42.42,4.32 v44.45,6.35

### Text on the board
Bottom: v03
tPlace: Reset | RED / 5V | TEMP | ST | WHT / SIG | ISP | RX | BLK / GND | TX | RED / E+ | LOAD CELL | BLK / E- | GND | OpenScale | WHT / A- | GND | 5V | GRN / A+ | RX | YLW / SHD | RATE | TX | DTR | B+ | B-
bPlace: 5V | SIG | GND | Ext Temp | RED | BLK | BLK | GND | FTDI | WHT | OpenScale | GND | GRN | 5V | RX | YLW | Load Cell | TX | GRN | DTR | B+ | B-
